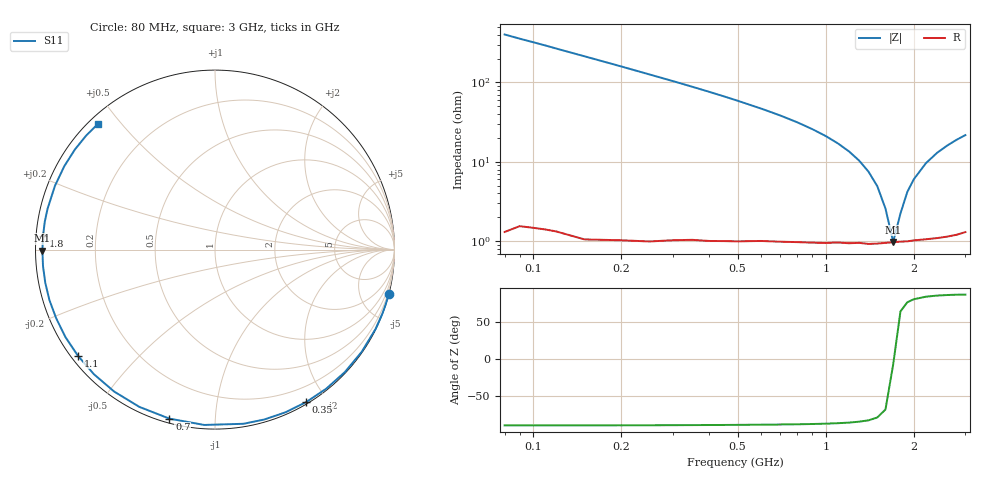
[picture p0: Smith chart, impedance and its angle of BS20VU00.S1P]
! SIEMENS Small Signal Semiconductors
! BB640
! Si Tuning Diode in SOD323
! VR = 20 V
! S-Parameters:  July  1993
# GHz  S  MA  R  50
!  f  S11
! GHz  MAG  ANG
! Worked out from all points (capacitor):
!   33 points, 80 MHz to 3 GHz, reference 50 ohm
!   read as one part to ground: C = 4.95 pF near 80 MHz
!   lowest |Z| = 982 mohm at 1.7 GHz (marker M1)
!   series resonance near 1.706 GHz, so ESL is about 1.8 nH
!   S11 on the Smith chart (normalised r, x): 80 MHz: 0.03, -8.03; 350 MHz: 0.02, -1.76; 700 MHz: 0.02, -0.77; 1.1 GHz: 0.02, -0.34; 1.8 GHz: 0.02, +0.04; 3 GHz: 0.03, +0.43
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0.08  0.9992 -14.2
0.15  0.9978 -26.4
0.2  0.9963 -34.9
0.25  0.9946 -43.3
0.3  0.9923 -51.3
0.35  0.9899 -59.1
0.4  0.9879 -66.6
0.45  0.9856 -73.8
0.5  0.9834 -80.7
0.6  0.9788 -93.5
0.7  0.9754 -105.1
0.8  0.9724 -115.7
0.9  0.9701 -125.4
1  0.9682 -134.2
1.1  0.966 -142.3
1.2  0.9654 -149.7
1.3  0.964 -156.6
1.4  0.9644 -163.0
1.5  0.9636 -168.9
1.6  0.9626 -174.5
1.7  0.9618 -179.7
1.8  0.9612 175.4
2  0.9603 166.4
2.2  0.9599 158.3
2.4  0.9597 151.0
2.6  0.9593 144.5
2.8  0.9586 138.5
3  0.957 133.1
